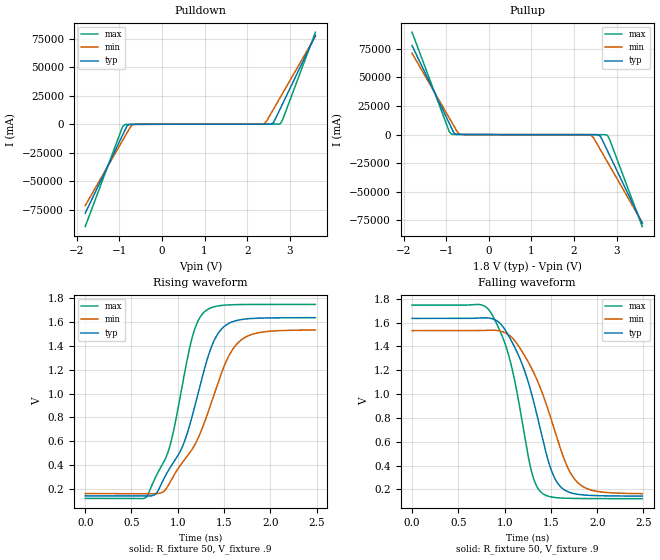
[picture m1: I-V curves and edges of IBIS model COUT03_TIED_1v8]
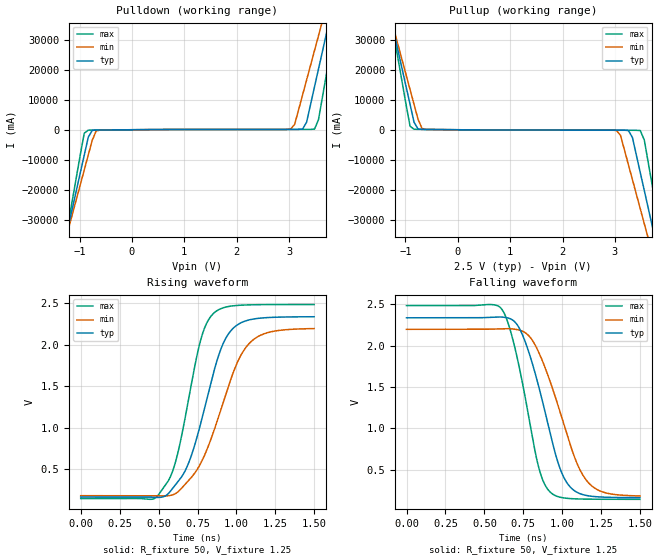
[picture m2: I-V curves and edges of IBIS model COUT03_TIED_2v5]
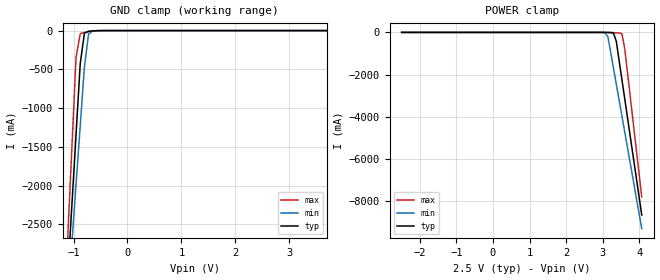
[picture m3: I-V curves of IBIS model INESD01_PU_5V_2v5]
|   This file is an IBIS representation of the   |
|   Integrated Device Technology, Inc   |
|   ICS83054I   |
|   4:1 Single-Ended Multiplexer   |
[IBIS Ver]   4.1
[File name]   83054i.ibs
[File Rev]   1.0
[Date]   2 Jun 2009 | Last modified
|   Mar 16 2006 | Generated
[Source]   Originated at Integrated Devices Technology, Inc.
[Disclaimer]
IDT hereby grants the user of this IBIS model a non-exclusive,
nontransferable license to use this IBIS model under the following terms.
Before using this IBIS model, the user should read this license.
If the user does not accept these terms,  the IBIS model should be
returned to IDT within 30 days.
   The user is granted this license only to use the IBIS model and
is not granted rights to sell, load, rent, lease or license the IBIS
model in whole or in part, or in modified form to anyone other than
user. User may modify the IBIS model to suit its specific
applications but rights to derivative works and such modifications
shall belong to IDT.
   This IBIS model is provided on an "AS IS" basis and IDT makes
absolutely no warranty with respect to the information contained
herein. IDT DISCLAIMS AND CUSTOMER WAIVES ALL WARRANTIES, EXPRESS
OR IMPLIED, INCLUDING WARRANTIES OF MERCHANTABILITY OR FITNESS FOR
A PARTICULAR PURPOSE. The entire risk as to quality and performance
is with the Customer. ACCORDINGLY, IN NO EVENT SHALL THE COMPANY BE
LIABLE FOR ANY DAMAGES, WHETHER IN CONTRACT OR TORT,INCLUDING ANY
LOST PROFITS OR OTHER INCIDENTAL, CONSEQUENTIAL, EXEMPLARY, OR
PUNITIVE DAMAGES ARISING OUT OF THE USE OR APPLICATION OF THE IBIS
model provided in this package. Further, IDT reserves the right to
make changes without notice to any product herein to improve
reliability, function, or design. IDT does not convey any license
under patent rights or any other intellectual property rights,
including those of third parties.
   IDT is not obligated to provide maintenance or support
for the licensed IBIS model.
[Copyright]   Copyright 2006 by Integrated Device Technology, Inc.
[Component]   ICS83054I
[Manufacturer] Integrated Devices Technology, Inc.
[Package]
|   TSSOP16   typ   min   max
R_pkg   58.65m   52.5m   64.8m
L_pkg   1.902nH   1.443nH   2.361nH
C_pkg   0.315pF   0.254pF   0.375pF
[Pin] signal_name   model_name   R_pin   L_pin   C_pin
1   Q   COUT03_TIED   64.8m   2.361n   0.375p
2   NC   NC   60.7m   2.054n   0.335p
3   OE   INESD01_PU_5V   56.6m   1.749n   0.294p
4   CLK3   INESD01_PD_NO_VD   52.5m   1.443n   0.254p
5   GND   GND   52.5m   1.443n   0.254p
6   NC   NC   56.6m   1.749n   0.294p
7   SEL1   INESD01_PD_5V   60.7m   2.054n   0.335p
8   CLK2   INESD01_PD_NO_VD   64.8m   2.361n   0.375p
9   SEL0   INESD01_PD_5V   64.8m   2.361n   0.375p
10   CLK1   INESD01_PD_NO_VD   60.7m   2.054n   0.335p
11   NC   NC   56.6m   1.749n   0.294p
12   VDD   POWER   52.5m   1.443n   0.254p
13   NC   NC   52.5m   1.443n   0.254p
14   CLK0   INESD01_PD_NO_VD   56.6m   1.749n   0.294p
15   NC   NC   60.7m   2.054n   0.335p
16   VDDO   POWER   64.8m   2.361n   0.375p
[Model Selector] COUT03_TIED
COUT03_TIED_1v8  Buffer selection for 1v8
COUT03_TIED_2v5  Buffer selection for 2v5
COUT03_TIED_3v3  Buffer selection for 3v3
[Model Selector] INESD01_PU_5V
INESD01_PU_5V_2v5  Buffer selection for 2v5
INESD01_PU_5V_3v3  Buffer selection for 3v3
[Model Selector] INESD01_PD_NO_VD
INESD01_PD_NO_VD_2v5  Buffer selection for 2v5
INESD01_PD_NO_VD_3v3  Buffer selection for 3v3
[Model Selector] INESD01_PD_5V
INESD01_PD_5V_2v5  Buffer selection for 2v5
INESD01_PD_5V_3v3  Buffer selection for 3v3
| Models and submodels in the file (9): COUT03_TIED_1v8 (Output), COUT03_TIED_2v5 (Output), INESD01_PU_5V_2v5 (Input), INESD01_PD_NO_VD_2v5 (Input), INESD01_PD_5V_2v5 (Input), COUT03_TIED_3v3 (Output), INESD01_PU_5V_3v3 (Input), INESD01_PD_NO_VD_3v3 (Input), INESD01_PD_5V_3v3 (Input)
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[Model] COUT03_TIED_1v8
Model_type   Output
Polarity   Non-Inverting
Vmeas = .9
Rref = 50
Cref = 0
Vref = .9
|   typ   min   max
C_comp   2pF   1.5pF   2.5pF
|   typ   min   max
[Voltage range]  1.8V   1.710V   1.890V
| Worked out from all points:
|   slope of the pulldown table from 0 to 0.27 V, typ, clamps not added: 10.3 ohm
|   slope of the pullup table from 0 to 0.27 V, typ, clamps not added: 11.9 ohm
|   rising waveform, R_fixture 50, V_fixture .9: 20-80 % time 370ps typ, 453ps min, 278ps max; typ from 0.143 V to 1.64 V
|   falling waveform, R_fixture 50, V_fixture .9: 20-80 % time 327ps typ, 389ps min, 257ps max; typ from 1.64 V to 0.143 V
[pulldown]
|Voltage   I (typ)   I (min)   I (max)
-1.8V     -77.88A    -71.2A     -89.55A
-927.3mV  -9.821A    -14.52A    -2.535A
-872.7mV  -5.567A    -10.98A    -279.7mA
-818.2mV  -1.447A    -7.441A    -119.4mA
-709.1mV  -98.56mA   -919.5mA   -92.65mA
-654.5mV  -74.81mA   -208.2mA   -85.34mA
2.4V      58.79mA    507.6mA    70.84mA
2.455V    61.02mA    2.637A     70.98mA
2.618V    1.414A     13.25A     71.57mA
2.782V    14.02A     23.86A     493.4mA
2.836V    18.27A     27.4A      4.385A
3.6V      77.78A     76.94A     80.46A
[pullup]
|Voltage   I (typ)   I (min)   I (max)
-1.8V     77.89A     71.2A      89.57A
-927.3mV  9.823A     14.53A     2.543A
-872.7mV  5.569A     10.98A     287mA
-818.2mV  1.45A      7.444A     126.9mA
-709.1mV  101.7mA    922.5mA    99.62mA
-654.5mV  77.73mA    211.3mA    91.37mA
2.4V      -60.59mA   -515mA     -72.08mA
2.455V    -64.65mA   -2.647A    -72.76mA
2.618V    -1.428A    -13.27A    -79.03mA
2.782V    -14.05A    -23.89A    -515mA
2.836V    -18.3A     -27.43A    -4.411A
3.6V      -77.85A    -77.01A    -80.54A
[Ramp]
|   typ   min   max
dV/dt_r   1.195/0.568n   1.097/0.672n   1.302/0.454n
dV/dt_f   1.198/0.499n   1.099/0.587n   1.305/0.4n
[Rising Waveform]
R_fixture = 50
V_fixture = .9
V_fixture_max = .945
V_fixture_min = .855
C_fixture = 0.0p
| Time   typ   min   max
0s        142.8mV    161.8mV    121.5mV
669.8ps   141.6mV    161.9mV    141.9mV
771.9ps   167.8mV    161.3mV    317mV
901.4ps   358.7mV    236.1mV    524.7mV
1.043ns   542.1mV    414.8mV    1.045V
1.17ns    851.2mV    551.4mV    1.508V
1.295ns   1.223V     771mV      1.689V
1.449ns   1.518V     1.122V     1.736V
1.678ns   1.619V     1.444V     1.746V
2.488ns   1.636V     1.533V     1.747V
[Falling Waveform]
R_fixture = 50
V_fixture = .9
V_fixture_max = .945
V_fixture_min = .855
C_fixture = 0.0p
| Time   typ   min   max
0s        1.636V     1.533V     1.747V
844.1ps   1.637V     1.538V     1.693V
1.021ns   1.52V      1.509V     1.386V
1.15ns    1.326V     1.405V     945.8mV
1.287ns   1.015V     1.223V     360mV
1.402ns   652.9mV    1.021V     170.3mV
1.559ns   269.5mV    650.9mV    130mV
1.673ns   183.5mV    397.7mV    124.9mV
1.783ns   159mV      262.2mV    123.1mV
2.488ns   143.1mV    163.6mV    121.5mV
[Model] COUT03_TIED_2v5
Model_type  Output
Polarity   Non-Inverting
Vmeas = 1.25
Rref = 50
Cref = 0
Vref = 1.25
|Variable  typ   min   max
C_comp   2p   1.5p   2.5p
[Voltage Range]   2.5   2.375   2.625
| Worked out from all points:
|   slope of the pulldown table from 0 to 0.375 V, typ, clamps not added: 8.25 ohm
|   slope of the pullup table from 0 to 0.375 V, typ, clamps not added: 8.09 ohm
|   rising waveform, R_fixture 50, V_fixture 1.25: 20-80 % time 193ps typ, 233ps min, 152ps max; typ from 0.163 V to 2.34 V
|   falling waveform, R_fixture 50, V_fixture 1.25: 20-80 % time 182ps typ, 215ps min, 147ps max; typ from 2.34 V to 0.164 V
| Open source, no load
|  Voltage   I(typ)   I(min)   I(max)
[Pullup]
-2.5V     132.6A     116.7A     159.5A
-1.288V   37.98A     37.97A     38.54A
-1.212V   32.07A     33.05A     30.99A
-909.1mV  8.434A     13.37A     1.158A
-833.3mV  2.525A     8.451A     173.9mA
-606.1mV  90.63mA    109.2mA    109.4mA
3.03V     -134.4mA   -266.8mA   -166.9mA
3.333V    -2.551A    -16.58A    -175.2mA
3.485V    -14.36A    -26.42A    -275mA
3.712V    -32.08A    -41.17A    -18.54A
3.864V    -43.9A     -51.01A    -33.65A
5V        -132.5A    -124.8A    -146.9A
[Pulldown]
-2.5V     -132.5A    -116.7A    -159.4A
-1.288V   -37.96A    -37.96A    -38.51A
-1.212V   -32.05A    -33.04A    -30.96A
-909.1mV  -8.418A    -13.36A    -1.131A
-833.3mV  -2.509A    -8.439A    -148.2mA
-606.1mV  -78.65mA   -99.19mA   -90.66mA
3.03V     104.5mA    238.1mA    123.5mA
3.333V    2.506A     16.54A     124.3mA
3.485V    14.31A     26.37A     211mA
3.712V    32.01A     41.11A     18.46A
3.864V    43.82A     50.94A     33.55A
5V        132.4A     124.7A     146.8A
[Ramp]
|   typ   min   max
dV/dt_r   1.742/0.307n   1.614/0.37n   1.879/0.24n
dV/dt_f   1.746/0.272n   1.616/0.322n   1.882/0.22n
R_load =   50.0000
[Rising Waveform]
R_fixture = 50
V_fixture = 1.25   | VCC_typ
V_fixture_max = 1.3125   | VCC_max
V_fixture_min = 1.1875   | VCC_min
C_fixture = 0.0p
| Time   typ   min   max
0s        162.8mV    179.2mV    144.2mV
459.5ps   160.6mV    180.1mV    137.1mV
546.5ps   180.2mV    176.8mV    312.4mV
614.1ps   322.8mV    210.7mV    623.9mV
696.7ps   592.1mV    370.8mV    1.384V
777.8ps   1.105V     597mV      2.106V
860.4ps   1.714V     990.7mV    2.39V
952ps     2.139V     1.519V     2.462V
1.087ns   2.301V     2.025V     2.48V
1.498ns   2.337V     2.194V     2.484V
[Falling Waveform]
R_fixture = 50
V_fixture = 1.25   | VCC_typ
V_fixture_max = 1.3125   | VCC_max
V_fixture_min = 1.1875   | VCC_min
C_fixture = 0.0p
| Time   typ   min   max
0s        2.337V     2.198V     2.484V
597.6ps   2.347V     2.205V     2.469V
671.2ps   2.321V     2.204V     2.155V
764.3ps   2.037V     2.154V     1.353V
833.3ps   1.616V     1.981V     651.8mV
878.4ps   1.287V     1.789V     360.6mV
968.5ps   612.6mV    1.304V     179.4mV
1.036ns   327.6mV    893.1mV    155.3mV
1.192ns   180.2mV    301.7mV    145.9mV
1.498ns   163.9mV    185mV      144.3mV
[Model] INESD01_PU_5V_2v5
Model_type   Input
Polarity   Non-Inverting
Vinl = .87V
Vinh = 1.62V
|   typ   min   max
C_comp   2pF   1.5pF   2.5pF
|   typ   min   max
[Voltage range]  2.5V   2.375V   2.625V
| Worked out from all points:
|   GND clamp passes 1 mA (typ) near -0.54 V on its own axis
[GND_clamp]
|Voltage   I(typ)   I(min)   I(max)
-1.572V   -8.64A     -8.058A    -9.677A
-1.108V   -3.163A    -3.501A    -2.677A
-1.031V   -2.251A    -2.743A    -1.511A
-953.6mV  -1.339A    -1.985A    -344.3mA
-876.3mV  -427.8mA   -1.227A    -39.97mA
-799mV    -34.67mA   -470.6mA   -24.26mA
-721.6mV  -8.956mA   -46.07mA   -15.49mA
-644.3mV  -3.769mA   -5.089mA   -8.163mA
5V        48.71uA    63.95uA    35.85uA
[POWER_clamp]
|Voltage   I(typ)   I(min)   I(max)
-2.5V     48.71uA    60.9uA     37.74uA
3.067V    -1.276mA   -19.03mA   -266.4uA
3.144V    -3.769mA   -203.7mA   -1.321mA
3.299V    -34.67mA   -1.694A    -10.77mA
3.376V    -427.8mA   -2.452A    -18.7mA
3.531V    -2.251A    -3.969A    -65.35mA
3.608V    -3.163A    -4.728A    -791.3mA
4.072V    -8.64A     -9.287A    -7.79A
